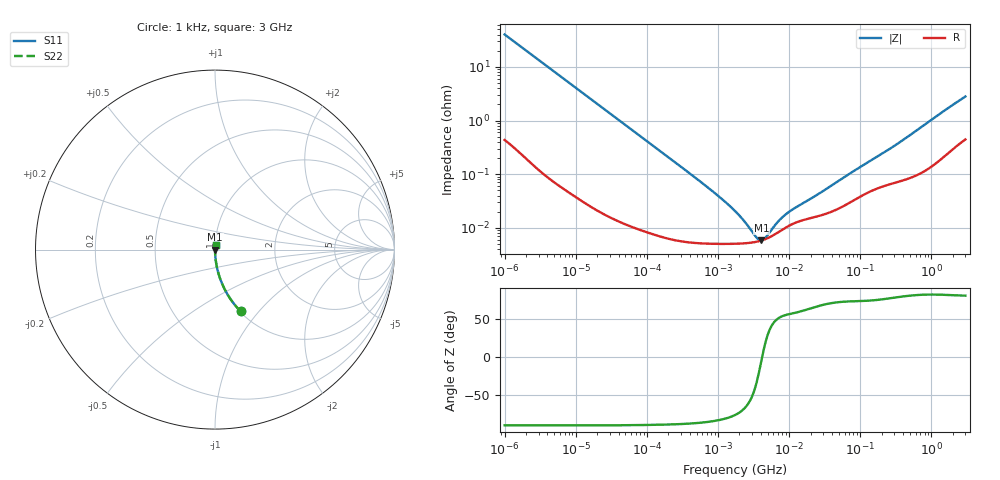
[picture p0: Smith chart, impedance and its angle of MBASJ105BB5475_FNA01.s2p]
! MBASJ105BB5475_FNA01  S-PARAMETER MODEL  ( Standard Model )
! Model Generated by TAIYO YUDEN Corporation (http://www.ty-top.com)
! Version 1.0
! TAIYO YUDEN Control No. 220601
! Copyright(c) 2013 TAIYO YUDEN CO.,LTD. All Rights Reserved.
! Product Description (link to TY-COMPAS)
! https://ds.yuden.co.jp/TYCOMPAS/or/detail?pn=MBASJ105BB5475MFNA01&u=M
! Products Name : Multilayer Ceramic Capacitors
! Characteristics :
!  Capacitance : 4.7 [uF] , Rated Voltage : 6.3 [V] , TCC : X5R
!  Case Size : 1.0 x 0.5 / 0.039 x 0.02 [mm/inch] , Thickness : 0.5 / 0.02 [mm/inch]
!  (Conditions: Temperature = 25 [degC] , DC Bias Voltage = 0 [V])
! External Node Assignments :
!  1  o---| |---o  2
! GND o---------o GND
! Frequency Range : 1kHz  -  3GHz  [ 401 STEP ]
# MHZ S RI R 50
! Freq[MHz].  S11 Real  S11 Imag  S21 Real  S21 Imag  S12 Real  S12 Imag  S22 Real  S22 Imag
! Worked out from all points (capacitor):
!   401 points, 1 kHz to 3 GHz, reference 50 ohm
!   read as one part in series: C = 3.93 uF near 1.077 kHz
!   lowest |Z| = 5.81 mohm at 4.083 MHz (marker M1)
!   series resonance near 4.163 MHz, so ESL is about 370 pH
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0.001  0.1427 -0.3444  0.8573 0.3444  0.8573 0.3444  0.1427 -0.3444
0.001685  0.0567 -0.2263  0.9433 0.2263  0.9433 0.2263  0.0567 -0.2263
0.00306  0.0185 -0.1303  0.9815 0.1303  0.9815 0.1303  0.0185 -0.1303
0.005768  0.00558 -0.0703  0.9944 0.0703  0.9944 0.0703  0.00558 -0.0703
0.01216  0.00145 -0.0336  0.9986 0.0336  0.9986 0.0336  0.00145 -0.0336
0.147855  7.77e-05 -0.0028  0.9999 0.0028  0.9999 0.0028  7.77e-05 -0.0028
0.791611  5.06e-05 -0.000508  0.9999 0.000508  0.9999 0.000508  5.06e-05 -0.000508
1.238299  5.01e-05 -0.000308  0.9999 0.000308  0.9999 0.000308  5.01e-05 -0.000308
1.732051  5.04e-05 -0.0002  0.9999 0.0002  0.9999 0.0002  5.04e-05 -0.0002
2.610246  5.2e-05 -9.75e-05  0.9999 9.75e-05  0.9999 9.75e-05  5.2e-05 -9.75e-05
2.812335  5.25e-05 -8.11e-05  0.9999 8.11e-05  0.9999 8.11e-05  5.25e-05 -8.11e-05
3.03007  5.32e-05 -6.51e-05  0.9999 6.51e-05  0.9999 6.51e-05  5.32e-05 -6.51e-05
4.083148  5.8e-05 -3.86e-06  0.9999 3.86e-06  0.9999 3.86e-06  5.8e-05 -3.86e-06
5.502215  6.83e-05 5.54e-05  0.9999 -5.54e-05  0.9999 -5.54e-05  6.83e-05 5.54e-05
5.928204  7.21e-05 7e-05  0.9999 -7e-05  0.9999 -7e-05  7.21e-05 7e-05
7.988506  9.22e-05 0.000126  0.9999 -0.000126  0.9999 -0.000126  9.22e-05 0.000126
9.625639  0.000107 0.00016  0.9999 -0.00016  0.9999 -0.00016  0.000107 0.00016
21.06097  0.000154 0.000328  0.9998 -0.000328  0.9998 -0.000328  0.000154 0.000328
80.61565  0.000325 0.00109  0.9997 -0.00109  0.9997 -0.00109  0.000325 0.00109
256.0921  0.000653 0.00286  0.9993 -0.00286  0.9993 -0.00286  0.000653 0.00286
1780.008  0.00286 0.0174  0.9971 -0.0174  0.9971 -0.0174  0.00286 0.0174
3000  0.00519 0.0275  0.9948 -0.0275  0.9948 -0.0275  0.00519 0.0275
